DATA_BLOCK "IMAC_VALVE_I/O"
TITLE =
AUTHOR : Hottendo
FAMILY : IMAC
VERSION : 0.2


  STRUCT
   VALVE_001_ACOM : WORD ;	//VALVE - Instance 001 : 'AUTO' Mode  Command Interface
   VALVE_001_STAT : WORD ;	//                       'AUTO' Mode  Status Interface
   VALVE_00l_OSSTAT : WORD ;	//                       OS Status Word
   VALVE_00l_OSALARM : WORD ;	//                       OS Alarm Word
   VALVE_001_OSCOM : WORD ;	//                       OS Command Interface
   VALVE_002_ACOM : WORD ;	//VALVE - Instance 002 : 'AUTO' Mode  Command Interface
   VALVE_002_STAT : WORD ;	//                       'AUTO' Mode  Status Interface
   VALVE_002_OSSTAT : WORD ;	//                       OS Status Word
   VALVE_002_OSALARM : WORD ;	//                       OS Alarm Word
   VALVE_002_OSCOM : WORD ;	//                       OS Command Interface
   VALVE_003_ACOM : WORD ;	//VALVE - Instance 003 : 'AUTO' Mode  Command Interface
   VALVE_003_STAT : WORD ;	//                       'AUTO' Mode  Status Interface
   VALVE_003_OSSTAT : WORD ;	//                       OS Status Word
   VALVE_003_OSALARM : WORD ;	//                       OS Alarm Word
   VALVE_003_OSCOM : WORD ;	//                       OS Command Interface
   VALVE_004_ACOM : WORD ;	//VALVE - Instance 004 : 'AUTO' Mode  Command Interface
   VALVE_004_STAT : WORD ;	//                       'AUTO' Mode  Status Interface
   VALVE_004_OSSTAT : WORD ;	//                       OS Status Word
   VALVE_004_OSALARM : WORD ;	//                       OS Alarm Word
   VALVE_004_OSCOM : WORD ;	//                       OS Command Interface
   VALVE_005_ACOM : WORD ;	//VALVE - Instance 005 : 'AUTO' Mode  Command Interface
   VALVE_005_STAT : WORD ;	//                       'AUTO' Mode  Status Interface
   VALVE_005_OSSTAT : WORD ;	//                       OS Status Word
   VALVE_005_OSALARM : WORD ;	//                       OS Alarm Word
   VALVE_005_OSCOM : WORD ;	//                       OS Command Interface
   VALVE_006_ACOM : WORD ;	//VALVE - Instance 006 : 'AUTO' Mode  Command Interface
   VALVE_006_STAT : WORD ;	//                       'AUTO' Mode  Status Interface
   VALVE_006_OSSTAT : WORD ;	//                       OS Status Word
   VALVE_006_OSALARM : WORD ;	//                       OS Alarm Word
   VALVE_006_OSCOM : WORD ;	//                       OS Command Interface
   VALVE_007_ACOM : WORD ;	//VALVE - Instance 007 : 'AUTO' Mode  Command Interface
   VALVE_007_STAT : WORD ;	//                       'AUTO' Mode  Status Interface
   VALVE_007_OSSTAT : WORD ;	//                       OS Status Word
   VALVE_007_OSALARM : WORD ;	//                       OS Alarm Word
   VALVE_007_OSCOM : WORD ;	//                       OS Command Interface
   VALVE_008_ACOM : WORD ;	//VALVE - Instance 008 : 'AUTO' Mode  Command Interface
   VALVE_008_STAT : WORD ;	//                       'AUTO' Mode  Status Interface
   VALVE_008_OSSTAT : WORD ;	//                       OS Status Word
   VALVE_008_OSALARM : WORD ;	//                       OS Alarm Word
   VALVE_008_OSCOM : WORD ;	//                       OS Command Interface
   VALVE_009_ACOM : WORD ;	//VALVE - Instance 009 : 'AUTO' Mode  Command Interface
   VALVE_009_STAT : WORD ;	//                       'AUTO' Mode  Status Interface
   VALVE_009_OSSTAT : WORD ;	//                       OS Status Word
   VALVE_009_OSALARM : WORD ;	//                       OS Alarm Word
   VALVE_009_OSCOM : WORD ;	//                       OS Command Interface
   VALVE_010_ACOM : WORD ;	//VALVE - Instance 010 : 'AUTO' Mode  Command Interface
   VALVE_010_STAT : WORD ;	//                       'AUTO' Mode  Status Interface
   VALVE_010_OSSTAT : WORD ;	//                       OS Status Word
   VALVE_010_OSALARM : WORD ;	//                       OS Alarm Word
   VALVE_010_OSCOM : WORD ;	//                       OS Command Interface
   VALVE_011_ACOM : WORD ;	//VALVE - Instance 011 : 'AUTO' Mode  Command Interface
   VALVE_011_STAT : WORD ;	//                       'AUTO' Mode  Status Interface
   VALVE_01l_OSSTAT : WORD ;	//                       OS Status Word
   VALVE_01l_OSALARM : WORD ;	//                       OS Alarm Word
   VALVE_011_OSCOM : WORD ;	//                       OS Command Interface
   VALVE_012_ACOM : WORD ;	//VALVE - Instance 012 : 'AUTO' Mode  Command Interface
   VALVE_012_STAT : WORD ;	//                       'AUTO' Mode  Status Interface
   VALVE_012_OSSTAT : WORD ;	//                       OS Status Word
   VALVE_012_OSALARM : WORD ;	//                       OS Alarm Word
   VALVE_012_OSCOM : WORD ;	//                       OS Command Interface
   VALVE_013_ACOM : WORD ;	//VALVE - Instance 013 : 'AUTO' Mode  Command Interface
   VALVE_013_STAT : WORD ;	//                       'AUTO' Mode  Status Interface
   VALVE_013_OSSTAT : WORD ;	//                       OS Status Word
   VALVE_013_OSALARM : WORD ;	//                       OS Alarm Word
   VALVE_013_OSCOM : WORD ;	//                       OS Command Interface
   VALVE_014_ACOM : WORD ;	//VALVE - Instance 014 : 'AUTO' Mode  Command Interface
   VALVE_014_STAT : WORD ;	//                       'AUTO' Mode  Status Interface
   VALVE_014_OSSTAT : WORD ;	//                       OS Status Word
   VALVE_014_OSALARM : WORD ;	//                       OS Alarm Word
   VALVE_014_OSCOM : WORD ;	//                       OS Command Interface
   VALVE_015_ACOM : WORD ;	//VALVE - Instance 015 : 'AUTO' Mode  Command Interface
   VALVE_015_STAT : WORD ;	//                       'AUTO' Mode  Status Interface
   VALVE_015_OSSTAT : WORD ;	//                       OS Status Word
   VALVE_015_OSALARM : WORD ;	//                       OS Alarm Word
   VALVE_015_OSCOM : WORD ;	//                       OS Command Interface
   VALVE_016_ACOM : WORD ;	//VALVE - Instance 016 : 'AUTO' Mode  Command Interface
   VALVE_016_STAT : WORD ;	//                       'AUTO' Mode  Status Interface
   VALVE_016_OSSTAT : WORD ;	//                       OS Status Word
   VALVE_016_OSALARM : WORD ;	//                       OS Alarm Word
   VALVE_016_OSCOM : WORD ;	//                       OS Command Interface
   VALVE_017_ACOM : WORD ;	//VALVE - Instance 017 : 'AUTO' Mode  Command Interface
   VALVE_017_STAT : WORD ;	//                       'AUTO' Mode  Status Interface
   VALVE_017_OSSTAT : WORD ;	//                       OS Status Word
   VALVE_017_OSALARM : WORD ;	//                       OS Alarm Word
   VALVE_017_OSCOM : WORD ;	//                       OS Command Interface
   VALVE_018_ACOM : WORD ;	//VALVE - Instance 018 : 'AUTO' Mode  Command Interface
   VALVE_018_STAT : WORD ;	//                       'AUTO' Mode  Status Interface
   VALVE_018_OSSTAT : WORD ;	//                       OS Status Word
   VALVE_018_OSALARM : WORD ;	//                       OS Alarm Word
   VALVE_018_OSCOM : WORD ;	//                       OS Command Interface
   VALVE_019_ACOM : WORD ;	//VALVE - Instance 019 : 'AUTO' Mode  Command Interface
   VALVE_019_STAT : WORD ;	//                       'AUTO' Mode  Status Interface
   VALVE_019_OSSTAT : WORD ;	//                       OS Status Word
   VALVE_019_OSALARM : WORD ;	//                       OS Alarm Word
   VALVE_019_OSCOM : WORD ;	//                       OS Command Interface
   VALVE_020_ACOM : WORD ;	//VALVE - Instance 020 : 'AUTO' Mode  Command Interface
   VALVE_020_STAT : WORD ;	//                       'AUTO' Mode  Status Interface
   VALVE_020_OSSTAT : WORD ;	//                       OS Status Word
   VALVE_020_OSALARM : WORD ;	//                       OS Alarm Word
   VALVE_020_OSCOM : WORD ;	//                       OS Command Interface
   VALVE_021_ACOM : WORD ;	//VALVE - Instance 021 : 'AUTO' Mode  Command Interface
   VALVE_021_STAT : WORD ;	//                       'AUTO' Mode  Status Interface
   VALVE_02l_OSSTAT : WORD ;	//                       OS Status Word
   VALVE_02l_OSALARM : WORD ;	//                       OS Alarm Word
   VALVE_021_OSCOM : WORD ;	//                       OS Command Interface
   VALVE_022_ACOM : WORD ;	//VALVE - Instance 022 : 'AUTO' Mode  Command Interface
   VALVE_022_STAT : WORD ;	//                       'AUTO' Mode  Status Interface
   VALVE_022_OSSTAT : WORD ;	//                       OS Status Word
   VALVE_022_OSALARM : WORD ;	//                       OS Alarm Word
   VALVE_022_OSCOM : WORD ;	//                       OS Command Interface
   VALVE_023_ACOM : WORD ;	//VALVE - Instance 023 : 'AUTO' Mode  Command Interface
   VALVE_023_STAT : WORD ;	//                       'AUTO' Mode  Status Interface
   VALVE_023_OSSTAT : WORD ;	//                       OS Status Word
   VALVE_023_OSALARM : WORD ;	//                       OS Alarm Word
   VALVE_023_OSCOM : WORD ;	//                       OS Command Interface
   VALVE_024_ACOM : WORD ;	//VALVE - Instance 024 : 'AUTO' Mode  Command Interface
   VALVE_024_STAT : WORD ;	//                       'AUTO' Mode  Status Interface
   VALVE_024_OSSTAT : WORD ;	//                       OS Status Word
   VALVE_024_OSALARM : WORD ;	//                       OS Alarm Word
   VALVE_024_OSCOM : WORD ;	//                       OS Command Interface
   VALVE_025_ACOM : WORD ;	//VALVE - Instance 025 : 'AUTO' Mode  Command Interface
   VALVE_025_STAT : WORD ;	//                       'AUTO' Mode  Status Interface
   VALVE_025_OSSTAT : WORD ;	//                       OS Status Word
   VALVE_025_OSALARM : WORD ;	//                       OS Alarm Word
   VALVE_025_OSCOM : WORD ;	//                       OS Command Interface
   VALVE_026_ACOM : WORD ;	//VALVE - Instance 026 : 'AUTO' Mode  Command Interface
   VALVE_026_STAT : WORD ;	//                       'AUTO' Mode  Status Interface
   VALVE_026_OSSTAT : WORD ;	//                       OS Status Word
   VALVE_026_OSALARM : WORD ;	//                       OS Alarm Word
   VALVE_026_OSCOM : WORD ;	//                       OS Command Interface
   VALVE_027_ACOM : WORD ;	//VALVE - Instance 027 : 'AUTO' Mode  Command Interface
   VALVE_027_STAT : WORD ;	//                       'AUTO' Mode  Status Interface
   VALVE_027_OSSTAT : WORD ;	//                       OS Status Word
   VALVE_027_OSALARM : WORD ;	//                       OS Alarm Word
   VALVE_027_OSCOM : WORD ;	//                       OS Command Interface
   VALVE_028_ACOM : WORD ;	//VALVE - Instance 028 : 'AUTO' Mode  Command Interface
   VALVE_028_STAT : WORD ;	//                       'AUTO' Mode  Status Interface
   VALVE_028_OSSTAT : WORD ;	//                       OS Status Word
   VALVE_028_OSALARM : WORD ;	//                       OS Alarm Word
   VALVE_028_OSCOM : WORD ;	//                       OS Command Interface
   VALVE_029_ACOM : WORD ;	//VALVE - Instance 029 : 'AUTO' Mode  Command Interface
   VALVE_029_STAT : WORD ;	//                       'AUTO' Mode  Status Interface
   VALVE_029_OSSTAT : WORD ;	//                       OS Status Word
   VALVE_029_OSALARM : WORD ;	//                       OS Alarm Word
   VALVE_029_OSCOM : WORD ;	//                       OS Command Interface
   VALVE_030_ACOM : WORD ;	//VALVE - Instance 030 : 'AUTO' Mode  Command Interface
   VALVE_030_STAT : WORD ;	//                       'AUTO' Mode  Status Interface
   VALVE_030_OSSTAT : WORD ;	//                       OS Status Word
   VALVE_030_OSALARM : WORD ;	//                       OS Alarm Word
   VALVE_030_OSCOM : WORD ;	//                       OS Command Interface
   VALVE_031_ACOM : WORD ;	//VALVE - Instance 031 : 'AUTO' Mode  Command Interface
   VALVE_031_STAT : WORD ;	//                       'AUTO' Mode  Status Interface
   VALVE_03l_OSSTAT : WORD ;	//                       OS Status Word
   VALVE_03l_OSALARM : WORD ;	//                       OS Alarm Word
   VALVE_031_OSCOM : WORD ;	//                       OS Command Interface
   VALVE_032_ACOM : WORD ;	//VALVE - Instance 032 : 'AUTO' Mode  Command Interface
   VALVE_032_STAT : WORD ;	//                       'AUTO' Mode  Status Interface
   VALVE_032_OSSTAT : WORD ;	//                       OS Status Word
   VALVE_032_OSALARM : WORD ;	//                       OS Alarm Word
   VALVE_032_OSCOM : WORD ;	//                       OS Command Interface
   VALVE_033_ACOM : WORD ;	//VALVE - Instance 033 : 'AUTO' Mode  Command Interface
   VALVE_033_STAT : WORD ;	//                       'AUTO' Mode  Status Interface
   VALVE_033_OSSTAT : WORD ;	//                       OS Status Word
   VALVE_033_OSALARM : WORD ;	//                       OS Alarm Word
   VALVE_033_OSCOM : WORD ;	//                       OS Command Interface
   VALVE_034_ACOM : WORD ;	//VALVE - Instance 034 : 'AUTO' Mode  Command Interface
   VALVE_034_STAT : WORD ;	//                       'AUTO' Mode  Status Interface
   VALVE_034_OSSTAT : WORD ;	//                       OS Status Word
   VALVE_034_OSALARM : WORD ;	//                       OS Alarm Word
   VALVE_034_OSCOM : WORD ;	//                       OS Command Interface
   VALVE_035_ACOM : WORD ;	//VALVE - Instance 035 : 'AUTO' Mode  Command Interface
   VALVE_035_STAT : WORD ;	//                       'AUTO' Mode  Status Interface
   VALVE_035_OSSTAT : WORD ;	//                       OS Status Word
   VALVE_035_OSALARM : WORD ;	//                       OS Alarm Word
   VALVE_035_OSCOM : WORD ;	//                       OS Command Interface
   VALVE_036_ACOM : WORD ;	//VALVE - Instance 036 : 'AUTO' Mode  Command Interface
   VALVE_036_STAT : WORD ;	//                       'AUTO' Mode  Status Interface
   VALVE_036_OSSTAT : WORD ;	//                       OS Status Word
   VALVE_036_OSALARM : WORD ;	//                       OS Alarm Word
   VALVE_036_OSCOM : WORD ;	//                       OS Command Interface
   VALVE_037_ACOM : WORD ;	//VALVE - Instance 037 : 'AUTO' Mode  Command Interface
   VALVE_037_STAT : WORD ;	//                       'AUTO' Mode  Status Interface
   VALVE_037_OSSTAT : WORD ;	//                       OS Status Word
   VALVE_037_OSALARM : WORD ;	//                       OS Alarm Word
   VALVE_037_OSCOM : WORD ;	//                       OS Command Interface
   VALVE_038_ACOM : WORD ;	//VALVE - Instance 038 : 'AUTO' Mode  Command Interface
   VALVE_038_STAT : WORD ;	//                       'AUTO' Mode  Status Interface
   VALVE_038_OSSTAT : WORD ;	//                       OS Status Word
   VALVE_038_OSALARM : WORD ;	//                       OS Alarm Word
   VALVE_038_OSCOM : WORD ;	//                       OS Command Interface
   VALVE_039_ACOM : WORD ;	//VALVE - Instance 039 : 'AUTO' Mode  Command Interface
   VALVE_039_STAT : WORD ;	//                       'AUTO' Mode  Status Interface
   VALVE_039_OSSTAT : WORD ;	//                       OS Status Word
   VALVE_039_OSALARM : WORD ;	//                       OS Alarm Word
   VALVE_039_OSCOM : WORD ;	//                       OS Command Interface
   VALVE_040_ACOM : WORD ;	//VALVE - Instance 040 : 'AUTO' Mode  Command Interface
   VALVE_040_STAT : WORD ;	//                       'AUTO' Mode  Status Interface
   VALVE_040_OSSTAT : WORD ;	//                       OS Status Word
   VALVE_040_OSALARM : WORD ;	//                       OS Alarm Word
   VALVE_040_OSCOM : WORD ;	//                       OS Command Interface
   VALVE_041_ACOM : WORD ;	//VALVE - Instance 041 : 'AUTO' Mode  Command Interface
   VALVE_041_STAT : WORD ;	//                       'AUTO' Mode  Status Interface
   VALVE_04l_OSSTAT : WORD ;	//                       OS Status Word
   VALVE_04l_OSALARM : WORD ;	//                       OS Alarm Word
   VALVE_041_OSCOM : WORD ;	//                       OS Command Interface
   VALVE_042_ACOM : WORD ;	//VALVE - Instance 042 : 'AUTO' Mode  Command Interface
   VALVE_042_STAT : WORD ;	//                       'AUTO' Mode  Status Interface
   VALVE_042_OSSTAT : WORD ;	//                       OS Status Word
   VALVE_042_OSALARM : WORD ;	//                       OS Alarm Word
   VALVE_042_OSCOM : WORD ;	//                       OS Command Interface
   VALVE_043_ACOM : WORD ;	//VALVE - Instance 043 : 'AUTO' Mode  Command Interface
   VALVE_043_STAT : WORD ;	//                       'AUTO' Mode  Status Interface
   VALVE_043_OSSTAT : WORD ;	//                       OS Status Word
   VALVE_043_OSALARM : WORD ;	//                       OS Alarm Word
   VALVE_043_OSCOM : WORD ;	//                       OS Command Interface
   VALVE_044_ACOM : WORD ;	//VALVE - Instance 044 : 'AUTO' Mode  Command Interface
   VALVE_044_STAT : WORD ;	//                       'AUTO' Mode  Status Interface
   VALVE_044_OSSTAT : WORD ;	//                       OS Status Word
   VALVE_044_OSALARM : WORD ;	//                       OS Alarm Word
   VALVE_044_OSCOM : WORD ;	//                       OS Command Interface
   VALVE_045_ACOM : WORD ;	//VALVE - Instance 045 : 'AUTO' Mode  Command Interface
   VALVE_045_STAT : WORD ;	//                       'AUTO' Mode  Status Interface
   VALVE_045_OSSTAT : WORD ;	//                       OS Status Word
   VALVE_045_OSALARM : WORD ;	//                       OS Alarm Word
   VALVE_045_OSCOM : WORD ;	//                       OS Command Interface
   VALVE_046_ACOM : WORD ;	//VALVE - Instance 046 : 'AUTO' Mode  Command Interface
   VALVE_046_STAT : WORD ;	//                       'AUTO' Mode  Status Interface
   VALVE_046_OSSTAT : WORD ;	//                       OS Status Word
   VALVE_046_OSALARM : WORD ;	//                       OS Alarm Word
   VALVE_046_OSCOM : WORD ;	//                       OS Command Interface
   VALVE_047_ACOM : WORD ;	//VALVE - Instance 047 : 'AUTO' Mode  Command Interface
   VALVE_047_STAT : WORD ;	//                       'AUTO' Mode  Status Interface
   VALVE_047_OSSTAT : WORD ;	//                       OS Status Word
   VALVE_047_OSALARM : WORD ;	//                       OS Alarm Word
   VALVE_047_OSCOM : WORD ;	//                       OS Command Interface
   VALVE_048_ACOM : WORD ;	//VALVE - Instance 048 : 'AUTO' Mode  Command Interface
   VALVE_048_STAT : WORD ;	//                       'AUTO' Mode  Status Interface
   VALVE_048_OSSTAT : WORD ;	//                       OS Status Word
   VALVE_048_OSALARM : WORD ;	//                       OS Alarm Word
   VALVE_048_OSCOM : WORD ;	//                       OS Command Interface
   VALVE_049_ACOM : WORD ;	//VALVE - Instance 049 : 'AUTO' Mode  Command Interface
   VALVE_049_STAT : WORD ;	//                       'AUTO' Mode  Status Interface
   VALVE_049_OSSTAT : WORD ;	//                       OS Status Word
   VALVE_049_OSALARM : WORD ;	//                       OS Alarm Word
   VALVE_049_OSCOM : WORD ;	//                       OS Command Interface
   VALVE_050_ACOM : WORD ;	//VALVE - Instance 050 : 'AUTO' Mode  Command Interface
   VALVE_050_STAT : WORD ;	//                       'AUTO' Mode  Status Interface
   VALVE_050_OSSTAT : WORD ;	//                       OS Status Word
   VALVE_050_OSALARM : WORD ;	//                       OS Alarm Word
   VALVE_050_OSCOM : WORD ;	//                       OS Command Interface
   VALVE_051_ACOM : WORD ;	//VALVE - Instance 051 : 'AUTO' Mode  Command Interface
   VALVE_051_STAT : WORD ;	//                       'AUTO' Mode  Status Interface
   VALVE_05l_OSSTAT : WORD ;	//                       OS Status Word
   VALVE_05l_OSALARM : WORD ;	//                       OS Alarm Word
   VALVE_051_OSCOM : WORD ;	//                       OS Command Interface
   VALVE_052_ACOM : WORD ;	//VALVE - Instance 052 : 'AUTO' Mode  Command Interface
   VALVE_052_STAT : WORD ;	//                       'AUTO' Mode  Status Interface
   VALVE_052_OSSTAT : WORD ;	//                       OS Status Word
   VALVE_052_OSALARM : WORD ;	//                       OS Alarm Word
   VALVE_052_OSCOM : WORD ;	//                       OS Command Interface
   VALVE_053_ACOM : WORD ;	//VALVE - Instance 053 : 'AUTO' Mode  Command Interface
   VALVE_053_STAT : WORD ;	//                       'AUTO' Mode  Status Interface
   VALVE_053_OSSTAT : WORD ;	//                       OS Status Word
   VALVE_053_OSALARM : WORD ;	//                       OS Alarm Word
   VALVE_053_OSCOM : WORD ;	//                       OS Command Interface
   VALVE_054_ACOM : WORD ;	//VALVE - Instance 054 : 'AUTO' Mode  Command Interface
   VALVE_054_STAT : WORD ;	//                       'AUTO' Mode  Status Interface
   VALVE_054_OSSTAT : WORD ;	//                       OS Status Word
   VALVE_054_OSALARM : WORD ;	//                       OS Alarm Word
   VALVE_054_OSCOM : WORD ;	//                       OS Command Interface
   VALVE_055_ACOM : WORD ;	//VALVE - Instance 055 : 'AUTO' Mode  Command Interface
   VALVE_055_STAT : WORD ;	//                       'AUTO' Mode  Status Interface
   VALVE_055_OSSTAT : WORD ;	//                       OS Status Word
   VALVE_055_OSALARM : WORD ;	//                       OS Alarm Word
   VALVE_055_OSCOM : WORD ;	//                       OS Command Interface
   VALVE_056_ACOM : WORD ;	//VALVE - Instance 056 : 'AUTO' Mode  Command Interface
   VALVE_056_STAT : WORD ;	//                       'AUTO' Mode  Status Interface
   VALVE_056_OSSTAT : WORD ;	//                       OS Status Word
   VALVE_056_OSALARM : WORD ;	//                       OS Alarm Word
   VALVE_056_OSCOM : WORD ;	//                       OS Command Interface
   VALVE_057_ACOM : WORD ;	//VALVE - Instance 057 : 'AUTO' Mode  Command Interface
   VALVE_057_STAT : WORD ;	//                       'AUTO' Mode  Status Interface
   VALVE_057_OSSTAT : WORD ;	//                       OS Status Word
   VALVE_057_OSALARM : WORD ;	//                       OS Alarm Word
   VALVE_057_OSCOM : WORD ;	//                       OS Command Interface
   VALVE_058_ACOM : WORD ;	//VALVE - Instance 058 : 'AUTO' Mode  Command Interface
   VALVE_058_STAT : WORD ;	//                       'AUTO' Mode  Status Interface
   VALVE_058_OSSTAT : WORD ;	//                       OS Status Word
   VALVE_058_OSALARM : WORD ;	//                       OS Alarm Word
   VALVE_058_OSCOM : WORD ;	//                       OS Command Interface
   VALVE_059_ACOM : WORD ;	//VALVE - Instance 059 : 'AUTO' Mode  Command Interface
   VALVE_059_STAT : WORD ;	//                       'AUTO' Mode  Status Interface
   VALVE_059_OSSTAT : WORD ;	//                       OS Status Word
   VALVE_059_OSALARM : WORD ;	//                       OS Alarm Word
   VALVE_059_OSCOM : WORD ;	//                       OS Command Interface
   VALVE_060_ACOM : WORD ;	//VALVE - Instance 060 : 'AUTO' Mode  Command Interface
   VALVE_060_STAT : WORD ;	//                       'AUTO' Mode  Status Interface
   VALVE_060_OSSTAT : WORD ;	//                       OS Status Word
   VALVE_060_OSALARM : WORD ;	//                       OS Alarm Word
   VALVE_060_OSCOM : WORD ;	//                       OS Command Interface
   VALVE_061_ACOM : WORD ;	//VALVE - Instance 061 : 'AUTO' Mode  Command Interface
   VALVE_061_STAT : WORD ;	//                       'AUTO' Mode  Status Interface
   VALVE_06l_OSSTAT : WORD ;	//                       OS Status Word
   VALVE_06l_OSALARM : WORD ;	//                       OS Alarm Word
   VALVE_061_OSCOM : WORD ;	//                       OS Command Interface
   VALVE_062_ACOM : WORD ;	//VALVE - Instance 062 : 'AUTO' Mode  Command Interface
   VALVE_062_STAT : WORD ;	//                       'AUTO' Mode  Status Interface
   VALVE_062_OSSTAT : WORD ;	//                       OS Status Word
   VALVE_062_OSALARM : WORD ;	//                       OS Alarm Word
   VALVE_062_OSCOM : WORD ;	//                       OS Command Interface
   VALVE_063_ACOM : WORD ;	//VALVE - Instance 063 : 'AUTO' Mode  Command Interface
   VALVE_063_STAT : WORD ;	//                       'AUTO' Mode  Status Interface
   VALVE_063_OSSTAT : WORD ;	//                       OS Status Word
   VALVE_063_OSALARM : WORD ;	//                       OS Alarm Word
   VALVE_063_OSCOM : WORD ;	//                       OS Command Interface
   VALVE_064_ACOM : WORD ;	//VALVE - Instance 064 : 'AUTO' Mode  Command Interface
   VALVE_064_STAT : WORD ;	//                       'AUTO' Mode  Status Interface
   VALVE_064_OSSTAT : WORD ;	//                       OS Status Word
   VALVE_064_OSALARM : WORD ;	//                       OS Alarm Word
   VALVE_064_OSCOM : WORD ;	//                       OS Command Interface
   VALVE_065_ACOM : WORD ;	//VALVE - Instance 065 : 'AUTO' Mode  Command Interface
   VALVE_065_STAT : WORD ;	//                       'AUTO' Mode  Status Interface
   VALVE_065_OSSTAT : WORD ;	//                       OS Status Word
   VALVE_065_OSALARM : WORD ;	//                       OS Alarm Word
   VALVE_065_OSCOM : WORD ;	//                       OS Command Interface
   VALVE_066_ACOM : WORD ;	//VALVE - Instance 066 : 'AUTO' Mode  Command Interface
   VALVE_066_STAT : WORD ;	//                       'AUTO' Mode  Status Interface
   VALVE_066_OSSTAT : WORD ;	//                       OS Status Word
   VALVE_066_OSALARM : WORD ;	//                       OS Alarm Word
   VALVE_066_OSCOM : WORD ;	//                       OS Command Interface
   VALVE_067_ACOM : WORD ;	//VALVE - Instance 067 : 'AUTO' Mode  Command Interface
   VALVE_067_STAT : WORD ;	//                       'AUTO' Mode  Status Interface
   VALVE_067_OSSTAT : WORD ;	//                       OS Status Word
   VALVE_067_OSALARM : WORD ;	//                       OS Alarm Word
   VALVE_067_OSCOM : WORD ;	//                       OS Command Interface
   VALVE_068_ACOM : WORD ;	//VALVE - Instance 068 : 'AUTO' Mode  Command Interface
   VALVE_068_STAT : WORD ;	//                       'AUTO' Mode  Status Interface
   VALVE_068_OSSTAT : WORD ;	//                       OS Status Word
   VALVE_068_OSALARM : WORD ;	//                       OS Alarm Word
   VALVE_068_OSCOM : WORD ;	//                       OS Command Interface
   VALVE_069_ACOM : WORD ;	//VALVE - Instance 069 : 'AUTO' Mode  Command Interface
   VALVE_069_STAT : WORD ;	//                       'AUTO' Mode  Status Interface
   VALVE_069_OSSTAT : WORD ;	//                       OS Status Word
   VALVE_069_OSALARM : WORD ;	//                       OS Alarm Word
   VALVE_069_OSCOM : WORD ;	//                       OS Command Interface
   VALVE_070_ACOM : WORD ;	//VALVE - Instance 070 : 'AUTO' Mode  Command Interface
   VALVE_070_STAT : WORD ;	//                       'AUTO' Mode  Status Interface
   VALVE_070_OSSTAT : WORD ;	//                       OS Status Word
   VALVE_070_OSALARM : WORD ;	//                       OS Alarm Word
   VALVE_070_OSCOM : WORD ;	//                       OS Command Interface
   VALVE_071_ACOM : WORD ;	//VALVE - Instance 071 : 'AUTO' Mode  Command Interface
   VALVE_071_STAT : WORD ;	//                       'AUTO' Mode  Status Interface
   VALVE_07l_OSSTAT : WORD ;	//                       OS Status Word
   VALVE_07l_OSALARM : WORD ;	//                       OS Alarm Word
   VALVE_071_OSCOM : WORD ;	//                       OS Command Interface
   VALVE_072_ACOM : WORD ;	//VALVE - Instance 072 : 'AUTO' Mode  Command Interface
   VALVE_072_STAT : WORD ;	//                       'AUTO' Mode  Status Interface
   VALVE_072_OSSTAT : WORD ;	//                       OS Status Word
   VALVE_072_OSALARM : WORD ;	//                       OS Alarm Word
   VALVE_072_OSCOM : WORD ;	//                       OS Command Interface
   VALVE_073_ACOM : WORD ;	//VALVE - Instance 073 : 'AUTO' Mode  Command Interface
   VALVE_073_STAT : WORD ;	//                       'AUTO' Mode  Status Interface
   VALVE_073_OSSTAT : WORD ;	//                       OS Status Word
   VALVE_073_OSALARM : WORD ;	//                       OS Alarm Word
   VALVE_073_OSCOM : WORD ;	//                       OS Command Interface
   VALVE_074_ACOM : WORD ;	//VALVE - Instance 074 : 'AUTO' Mode  Command Interface
   VALVE_074_STAT : WORD ;	//                       'AUTO' Mode  Status Interface
   VALVE_074_OSSTAT : WORD ;	//                       OS Status Word
   VALVE_074_OSALARM : WORD ;	//                       OS Alarm Word
   VALVE_074_OSCOM : WORD ;	//                       OS Command Interface
   VALVE_075_ACOM : WORD ;	//VALVE - Instance 075 : 'AUTO' Mode  Command Interface
   VALVE_075_STAT : WORD ;	//                       'AUTO' Mode  Status Interface
   VALVE_075_OSSTAT : WORD ;	//                       OS Status Word
   VALVE_075_OSALARM : WORD ;	//                       OS Alarm Word
   VALVE_075_OSCOM : WORD ;	//                       OS Command Interface
   VALVE_076_ACOM : WORD ;	//VALVE - Instance 076 : 'AUTO' Mode  Command Interface
   VALVE_076_STAT : WORD ;	//                       'AUTO' Mode  Status Interface
   VALVE_076_OSSTAT : WORD ;	//                       OS Status Word
   VALVE_076_OSALARM : WORD ;	//                       OS Alarm Word
   VALVE_076_OSCOM : WORD ;	//                       OS Command Interface
   VALVE_077_ACOM : WORD ;	//VALVE - Instance 077 : 'AUTO' Mode  Command Interface
   VALVE_077_STAT : WORD ;	//                       'AUTO' Mode  Status Interface
   VALVE_077_OSSTAT : WORD ;	//                       OS Status Word
   VALVE_077_OSALARM : WORD ;	//                       OS Alarm Word
   VALVE_077_OSCOM : WORD ;	//                       OS Command Interface
   VALVE_078_ACOM : WORD ;	//VALVE - Instance 078 : 'AUTO' Mode  Command Interface
   VALVE_078_STAT : WORD ;	//                       'AUTO' Mode  Status Interface
   VALVE_078_OSSTAT : WORD ;	//                       OS Status Word
   VALVE_078_OSALARM : WORD ;	//                       OS Alarm Word
   VALVE_078_OSCOM : WORD ;	//                       OS Command Interface
   VALVE_079_ACOM : WORD ;	//VALVE - Instance 079 : 'AUTO' Mode  Command Interface
   VALVE_079_STAT : WORD ;	//                       'AUTO' Mode  Status Interface
   VALVE_079_OSSTAT : WORD ;	//                       OS Status Word
   VALVE_079_OSALARM : WORD ;	//                       OS Alarm Word
   VALVE_079_OSCOM : WORD ;	//                       OS Command Interface
   VALVE_080_ACOM : WORD ;	//VALVE - Instance 080 : 'AUTO' Mode  Command Interface
   VALVE_080_STAT : WORD ;	//                       'AUTO' Mode  Status Interface
   VALVE_080_OSSTAT : WORD ;	//                       OS Status Word
   VALVE_080_OSALARM : WORD ;	//                       OS Alarm Word
   VALVE_080_OSCOM : WORD ;	//                       OS Command Interface
   VALVE_081_ACOM : WORD ;	//VALVE - Instance 081 : 'AUTO' Mode  Command Interface
   VALVE_081_STAT : WORD ;	//                       'AUTO' Mode  Status Interface
   VALVE_08l_OSSTAT : WORD ;	//                       OS Status Word
   VALVE_08l_OSALARM : WORD ;	//                       OS Alarm Word
   VALVE_081_OSCOM : WORD ;	//                       OS Command Interface
   VALVE_082_ACOM : WORD ;	//VALVE - Instance 082 : 'AUTO' Mode  Command Interface
   VALVE_082_STAT : WORD ;	//                       'AUTO' Mode  Status Interface
   VALVE_082_OSSTAT : WORD ;	//                       OS Status Word
   VALVE_082_OSALARM : WORD ;	//                       OS Alarm Word
   VALVE_082_OSCOM : WORD ;	//                       OS Command Interface
   VALVE_083_ACOM : WORD ;	//VALVE - Instance 083 : 'AUTO' Mode  Command Interface
   VALVE_083_STAT : WORD ;	//                       'AUTO' Mode  Status Interface
   VALVE_083_OSSTAT : WORD ;	//                       OS Status Word
   VALVE_083_OSALARM : WORD ;	//                       OS Alarm Word
   VALVE_083_OSCOM : WORD ;	//                       OS Command Interface
   VALVE_084_ACOM : WORD ;	//VALVE - Instance 084 : 'AUTO' Mode  Command Interface
   VALVE_084_STAT : WORD ;	//                       'AUTO' Mode  Status Interface
   VALVE_084_OSSTAT : WORD ;	//                       OS Status Word
   VALVE_084_OSALARM : WORD ;	//                       OS Alarm Word
   VALVE_084_OSCOM : WORD ;	//                       OS Command Interface
   VALVE_085_ACOM : WORD ;	//VALVE - Instance 085 : 'AUTO' Mode  Command Interface
   VALVE_085_STAT : WORD ;	//                       'AUTO' Mode  Status Interface
   VALVE_085_OSSTAT : WORD ;	//                       OS Status Word
   VALVE_085_OSALARM : WORD ;	//                       OS Alarm Word
   VALVE_085_OSCOM : WORD ;	//                       OS Command Interface
   VALVE_086_ACOM : WORD ;	//VALVE - Instance 086 : 'AUTO' Mode  Command Interface
   VALVE_086_STAT : WORD ;	//                       'AUTO' Mode  Status Interface
   VALVE_086_OSSTAT : WORD ;	//                       OS Status Word
   VALVE_086_OSALARM : WORD ;	//                       OS Alarm Word
   VALVE_086_OSCOM : WORD ;	//                       OS Command Interface
   VALVE_087_ACOM : WORD ;	//VALVE - Instance 087 : 'AUTO' Mode  Command Interface
   VALVE_087_STAT : WORD ;	//                       'AUTO' Mode  Status Interface
   VALVE_087_OSSTAT : WORD ;	//                       OS Status Word
   VALVE_087_OSALARM : WORD ;	//                       OS Alarm Word
   VALVE_087_OSCOM : WORD ;	//                       OS Command Interface
   VALVE_088_ACOM : WORD ;	//VALVE - Instance 088 : 'AUTO' Mode  Command Interface
   VALVE_088_STAT : WORD ;	//                       'AUTO' Mode  Status Interface
   VALVE_088_OSSTAT : WORD ;	//                       OS Status Word
   VALVE_088_OSALARM : WORD ;	//                       OS Alarm Word
   VALVE_088_OSCOM : WORD ;	//                       OS Command Interface
   VALVE_089_ACOM : WORD ;	//VALVE - Instance 089 : 'AUTO' Mode  Command Interface
   VALVE_089_STAT : WORD ;	//                       'AUTO' Mode  Status Interface
   VALVE_089_OSSTAT : WORD ;	//                       OS Status Word
   VALVE_089_OSALARM : WORD ;	//                       OS Alarm Word
   VALVE_089_OSCOM : WORD ;	//                       OS Command Interface
   VALVE_090_ACOM : WORD ;	//VALVE - Instance 090 : 'AUTO' Mode  Command Interface
   VALVE_090_STAT : WORD ;	//                       'AUTO' Mode  Status Interface
   VALVE_090_OSSTAT : WORD ;	//                       OS Status Word
   VALVE_090_OSALARM : WORD ;	//                       OS Alarm Word
   VALVE_090_OSCOM : WORD ;	//                       OS Command Interface
   VALVE_091_ACOM : WORD ;	//VALVE - Instance 091 : 'AUTO' Mode  Command Interface
   VALVE_091_STAT : WORD ;	//                       'AUTO' Mode  Status Interface
   VALVE_09l_OSSTAT : WORD ;	//                       OS Status Word
   VALVE_09l_OSALARM : WORD ;	//                       OS Alarm Word
   VALVE_091_OSCOM : WORD ;	//                       OS Command Interface
   VALVE_092_ACOM : WORD ;	//VALVE - Instance 092 : 'AUTO' Mode  Command Interface
   VALVE_092_STAT : WORD ;	//                       'AUTO' Mode  Status Interface
   VALVE_092_OSSTAT : WORD ;	//                       OS Status Word
   VALVE_092_OSALARM : WORD ;	//                       OS Alarm Word
   VALVE_092_OSCOM : WORD ;	//                       OS Command Interface
   VALVE_093_ACOM : WORD ;	//VALVE - Instance 093 : 'AUTO' Mode  Command Interface
   VALVE_093_STAT : WORD ;	//                       'AUTO' Mode  Status Interface
   VALVE_093_OSSTAT : WORD ;	//                       OS Status Word
   VALVE_093_OSALARM : WORD ;	//                       OS Alarm Word
   VALVE_093_OSCOM : WORD ;	//                       OS Command Interface
   VALVE_094_ACOM : WORD ;	//VALVE - Instance 094 : 'AUTO' Mode  Command Interface
   VALVE_094_STAT : WORD ;	//                       'AUTO' Mode  Status Interface
   VALVE_094_OSSTAT : WORD ;	//                       OS Status Word
   VALVE_094_OSALARM : WORD ;	//                       OS Alarm Word
   VALVE_094_OSCOM : WORD ;	//                       OS Command Interface
   VALVE_095_ACOM : WORD ;	//VALVE - Instance 095 : 'AUTO' Mode  Command Interface
   VALVE_095_STAT : WORD ;	//                       'AUTO' Mode  Status Interface
   VALVE_095_OSSTAT : WORD ;	//                       OS Status Word
   VALVE_095_OSALARM : WORD ;	//                       OS Alarm Word
   VALVE_095_OSCOM : WORD ;	//                       OS Command Interface
   VALVE_096_ACOM : WORD ;	//VALVE - Instance 096 : 'AUTO' Mode  Command Interface
   VALVE_096_STAT : WORD ;	//                       'AUTO' Mode  Status Interface
   VALVE_096_OSSTAT : WORD ;	//                       OS Status Word
   VALVE_096_OSALARM : WORD ;	//                       OS Alarm Word
   VALVE_096_OSCOM : WORD ;	//                       OS Command Interface
   VALVE_097_ACOM : WORD ;	//VALVE - Instance 097 : 'AUTO' Mode  Command Interface
   VALVE_097_STAT : WORD ;	//                       'AUTO' Mode  Status Interface
   VALVE_097_OSSTAT : WORD ;	//                       OS Status Word
   VALVE_097_OSALARM : WORD ;	//                       OS Alarm Word
   VALVE_097_OSCOM : WORD ;	//                       OS Command Interface
   VALVE_098_ACOM : WORD ;	//VALVE - Instance 098 : 'AUTO' Mode  Command Interface
   VALVE_098_STAT : WORD ;	//                       'AUTO' Mode  Status Interface
   VALVE_098_OSSTAT : WORD ;	//                       OS Status Word
   VALVE_098_OSALARM : WORD ;	//                       OS Alarm Word
   VALVE_098_OSCOM : WORD ;	//                       OS Command Interface
   VALVE_099_ACOM : WORD ;	//VALVE - Instance 099 : 'AUTO' Mode  Command Interface
   VALVE_099_STAT : WORD ;	//                       'AUTO' Mode  Status Interface
   VALVE_099_OSSTAT : WORD ;	//                       OS Status Word
   VALVE_099_OSALARM : WORD ;	//                       OS Alarm Word
   VALVE_099_OSCOM : WORD ;	//                       OS Command Interface
   VALVE_100_ACOM : WORD ;	//VALVE - Instance 100 : 'AUTO' Mode  Command Interface
   VALVE_100_STAT : WORD ;	//                       'AUTO' Mode  Status Interface
   VALVE_100_OSSTAT : WORD ;	//                       OS Status Word
   VALVE_100_OSALARM : WORD ;	//                       OS Alarm Word
   VALVE_100_OSCOM : WORD ;	//                       OS Command Interface
   VALVE_100_ACOM1 : WORD ;	//VALVE - Instance 100 : 'AUTO' Mode  Command Interface
   VALVE_100_STAT1 : WORD ;	//                       'AUTO' Mode  Status Interface
   VALVE_100_OSSTAT1 : WORD ;	//                       OS Status Word
   VALVE_100_OSALARM1 : WORD ;	//                       OS Alarm Word
   VALVE_100_OSCOM1 : WORD ;	//                       OS Command Interface
  END_STRUCT ;
BEGIN
   VALVE_001_ACOM := W#16#0;
   VALVE_001_STAT := W#16#0;
   VALVE_00l_OSSTAT := W#16#0;
   VALVE_00l_OSALARM := W#16#0;
   VALVE_001_OSCOM := W#16#0;
   VALVE_002_ACOM := W#16#0;
   VALVE_002_STAT := W#16#0;
   VALVE_002_OSSTAT := W#16#0;
   VALVE_002_OSALARM := W#16#0;
   VALVE_002_OSCOM := W#16#0;
   VALVE_003_ACOM := W#16#0;
   VALVE_003_STAT := W#16#0;
   VALVE_003_OSSTAT := W#16#0;
   VALVE_003_OSALARM := W#16#0;
   VALVE_003_OSCOM := W#16#0;
   VALVE_004_ACOM := W#16#0;
   VALVE_004_STAT := W#16#0;
   VALVE_004_OSSTAT := W#16#0;
   VALVE_004_OSALARM := W#16#0;
   VALVE_004_OSCOM := W#16#0;
   VALVE_005_ACOM := W#16#0;
   VALVE_005_STAT := W#16#0;
   VALVE_005_OSSTAT := W#16#0;
   VALVE_005_OSALARM := W#16#0;
   VALVE_005_OSCOM := W#16#0;
   VALVE_006_ACOM := W#16#0;
   VALVE_006_STAT := W#16#0;
   VALVE_006_OSSTAT := W#16#0;
   VALVE_006_OSALARM := W#16#0;
   VALVE_006_OSCOM := W#16#0;
   VALVE_007_ACOM := W#16#0;
   VALVE_007_STAT := W#16#0;
   VALVE_007_OSSTAT := W#16#0;
   VALVE_007_OSALARM := W#16#0;
   VALVE_007_OSCOM := W#16#0;
   VALVE_008_ACOM := W#16#0;
   VALVE_008_STAT := W#16#0;
   VALVE_008_OSSTAT := W#16#0;
   VALVE_008_OSALARM := W#16#0;
   VALVE_008_OSCOM := W#16#0;
   VALVE_009_ACOM := W#16#0;
   VALVE_009_STAT := W#16#0;
   VALVE_009_OSSTAT := W#16#0;
   VALVE_009_OSALARM := W#16#0;
   VALVE_009_OSCOM := W#16#0;
   VALVE_010_ACOM := W#16#0;
   VALVE_010_STAT := W#16#0;
   VALVE_010_OSSTAT := W#16#0;
   VALVE_010_OSALARM := W#16#0;
   VALVE_010_OSCOM := W#16#0;
   VALVE_011_ACOM := W#16#0;
   VALVE_011_STAT := W#16#0;
   VALVE_01l_OSSTAT := W#16#0;
   VALVE_01l_OSALARM := W#16#0;
   VALVE_011_OSCOM := W#16#0;
   VALVE_012_ACOM := W#16#0;
   VALVE_012_STAT := W#16#0;
   VALVE_012_OSSTAT := W#16#0;
   VALVE_012_OSALARM := W#16#0;
   VALVE_012_OSCOM := W#16#0;
   VALVE_013_ACOM := W#16#0;
   VALVE_013_STAT := W#16#0;
   VALVE_013_OSSTAT := W#16#0;
   VALVE_013_OSALARM := W#16#0;
   VALVE_013_OSCOM := W#16#0;
   VALVE_014_ACOM := W#16#0;
   VALVE_014_STAT := W#16#0;
   VALVE_014_OSSTAT := W#16#0;
   VALVE_014_OSALARM := W#16#0;
   VALVE_014_OSCOM := W#16#0;
   VALVE_015_ACOM := W#16#0;
   VALVE_015_STAT := W#16#0;
   VALVE_015_OSSTAT := W#16#0;
   VALVE_015_OSALARM := W#16#0;
   VALVE_015_OSCOM := W#16#0;
   VALVE_016_ACOM := W#16#0;
   VALVE_016_STAT := W#16#0;
   VALVE_016_OSSTAT := W#16#0;
   VALVE_016_OSALARM := W#16#0;
   VALVE_016_OSCOM := W#16#0;
   VALVE_017_ACOM := W#16#0;
   VALVE_017_STAT := W#16#0;
   VALVE_017_OSSTAT := W#16#0;
   VALVE_017_OSALARM := W#16#0;
   VALVE_017_OSCOM := W#16#0;
   VALVE_018_ACOM := W#16#0;
   VALVE_018_STAT := W#16#0;
   VALVE_018_OSSTAT := W#16#0;
   VALVE_018_OSALARM := W#16#0;
   VALVE_018_OSCOM := W#16#0;
   VALVE_019_ACOM := W#16#0;
   VALVE_019_STAT := W#16#0;
   VALVE_019_OSSTAT := W#16#0;
   VALVE_019_OSALARM := W#16#0;
   VALVE_019_OSCOM := W#16#0;
   VALVE_020_ACOM := W#16#0;
   VALVE_020_STAT := W#16#0;
   VALVE_020_OSSTAT := W#16#0;
   VALVE_020_OSALARM := W#16#0;
   VALVE_020_OSCOM := W#16#0;
   VALVE_021_ACOM := W#16#0;
   VALVE_021_STAT := W#16#0;
   VALVE_02l_OSSTAT := W#16#0;
   VALVE_02l_OSALARM := W#16#0;
   VALVE_021_OSCOM := W#16#0;
   VALVE_022_ACOM := W#16#0;
   VALVE_022_STAT := W#16#0;
   VALVE_022_OSSTAT := W#16#0;
   VALVE_022_OSALARM := W#16#0;
   VALVE_022_OSCOM := W#16#0;
   VALVE_023_ACOM := W#16#0;
   VALVE_023_STAT := W#16#0;
   VALVE_023_OSSTAT := W#16#0;
   VALVE_023_OSALARM := W#16#0;
   VALVE_023_OSCOM := W#16#0;
   VALVE_024_ACOM := W#16#0;
   VALVE_024_STAT := W#16#0;
   VALVE_024_OSSTAT := W#16#0;
   VALVE_024_OSALARM := W#16#0;
   VALVE_024_OSCOM := W#16#0;
   VALVE_025_ACOM := W#16#0;
   VALVE_025_STAT := W#16#0;
   VALVE_025_OSSTAT := W#16#0;
   VALVE_025_OSALARM := W#16#0;
   VALVE_025_OSCOM := W#16#0;
   VALVE_026_ACOM := W#16#0;
   VALVE_026_STAT := W#16#0;
   VALVE_026_OSSTAT := W#16#0;
   VALVE_026_OSALARM := W#16#0;
   VALVE_026_OSCOM := W#16#0;
   VALVE_027_ACOM := W#16#0;
   VALVE_027_STAT := W#16#0;
   VALVE_027_OSSTAT := W#16#0;
   VALVE_027_OSALARM := W#16#0;
   VALVE_027_OSCOM := W#16#0;
   VALVE_028_ACOM := W#16#0;
   VALVE_028_STAT := W#16#0;
   VALVE_028_OSSTAT := W#16#0;
   VALVE_028_OSALARM := W#16#0;
   VALVE_028_OSCOM := W#16#0;
   VALVE_029_ACOM := W#16#0;
   VALVE_029_STAT := W#16#0;
   VALVE_029_OSSTAT := W#16#0;
   VALVE_029_OSALARM := W#16#0;
   VALVE_029_OSCOM := W#16#0;
   VALVE_030_ACOM := W#16#0;
   VALVE_030_STAT := W#16#0;
   VALVE_030_OSSTAT := W#16#0;
   VALVE_030_OSALARM := W#16#0;
   VALVE_030_OSCOM := W#16#0;
   VALVE_031_ACOM := W#16#0;
   VALVE_031_STAT := W#16#0;
   VALVE_03l_OSSTAT := W#16#0;
   VALVE_03l_OSALARM := W#16#0;
   VALVE_031_OSCOM := W#16#0;
   VALVE_032_ACOM := W#16#0;
   VALVE_032_STAT := W#16#0;
   VALVE_032_OSSTAT := W#16#0;
   VALVE_032_OSALARM := W#16#0;
   VALVE_032_OSCOM := W#16#0;
   VALVE_033_ACOM := W#16#0;
   VALVE_033_STAT := W#16#0;
   VALVE_033_OSSTAT := W#16#0;
   VALVE_033_OSALARM := W#16#0;
   VALVE_033_OSCOM := W#16#0;
   VALVE_034_ACOM := W#16#0;
   VALVE_034_STAT := W#16#0;
   VALVE_034_OSSTAT := W#16#0;
   VALVE_034_OSALARM := W#16#0;
   VALVE_034_OSCOM := W#16#0;
   VALVE_035_ACOM := W#16#0;
   VALVE_035_STAT := W#16#0;
   VALVE_035_OSSTAT := W#16#0;
   VALVE_035_OSALARM := W#16#0;
   VALVE_035_OSCOM := W#16#0;
   VALVE_036_ACOM := W#16#0;
   VALVE_036_STAT := W#16#0;
   VALVE_036_OSSTAT := W#16#0;
   VALVE_036_OSALARM := W#16#0;
   VALVE_036_OSCOM := W#16#0;
   VALVE_037_ACOM := W#16#0;
   VALVE_037_STAT := W#16#0;
   VALVE_037_OSSTAT := W#16#0;
   VALVE_037_OSALARM := W#16#0;
   VALVE_037_OSCOM := W#16#0;
   VALVE_038_ACOM := W#16#0;
   VALVE_038_STAT := W#16#0;
   VALVE_038_OSSTAT := W#16#0;
   VALVE_038_OSALARM := W#16#0;
   VALVE_038_OSCOM := W#16#0;
   VALVE_039_ACOM := W#16#0;
   VALVE_039_STAT := W#16#0;
   VALVE_039_OSSTAT := W#16#0;
   VALVE_039_OSALARM := W#16#0;
   VALVE_039_OSCOM := W#16#0;
   VALVE_040_ACOM := W#16#0;
   VALVE_040_STAT := W#16#0;
   VALVE_040_OSSTAT := W#16#0;
   VALVE_040_OSALARM := W#16#0;
   VALVE_040_OSCOM := W#16#0;
   VALVE_041_ACOM := W#16#0;
   VALVE_041_STAT := W#16#0;
   VALVE_04l_OSSTAT := W#16#0;
   VALVE_04l_OSALARM := W#16#0;
   VALVE_041_OSCOM := W#16#0;
   VALVE_042_ACOM := W#16#0;
   VALVE_042_STAT := W#16#0;
   VALVE_042_OSSTAT := W#16#0;
   VALVE_042_OSALARM := W#16#0;
   VALVE_042_OSCOM := W#16#0;
   VALVE_043_ACOM := W#16#0;
   VALVE_043_STAT := W#16#0;
   VALVE_043_OSSTAT := W#16#0;
   VALVE_043_OSALARM := W#16#0;
   VALVE_043_OSCOM := W#16#0;
   VALVE_044_ACOM := W#16#0;
   VALVE_044_STAT := W#16#0;
   VALVE_044_OSSTAT := W#16#0;
   VALVE_044_OSALARM := W#16#0;
   VALVE_044_OSCOM := W#16#0;
   VALVE_045_ACOM := W#16#0;
   VALVE_045_STAT := W#16#0;
   VALVE_045_OSSTAT := W#16#0;
   VALVE_045_OSALARM := W#16#0;
   VALVE_045_OSCOM := W#16#0;
   VALVE_046_ACOM := W#16#0;
   VALVE_046_STAT := W#16#0;
   VALVE_046_OSSTAT := W#16#0;
   VALVE_046_OSALARM := W#16#0;
   VALVE_046_OSCOM := W#16#0;
   VALVE_047_ACOM := W#16#0;
   VALVE_047_STAT := W#16#0;
   VALVE_047_OSSTAT := W#16#0;
   VALVE_047_OSALARM := W#16#0;
   VALVE_047_OSCOM := W#16#0;
   VALVE_048_ACOM := W#16#0;
   VALVE_048_STAT := W#16#0;
   VALVE_048_OSSTAT := W#16#0;
   VALVE_048_OSALARM := W#16#0;
   VALVE_048_OSCOM := W#16#0;
   VALVE_049_ACOM := W#16#0;
   VALVE_049_STAT := W#16#0;
   VALVE_049_OSSTAT := W#16#0;
   VALVE_049_OSALARM := W#16#0;
   VALVE_049_OSCOM := W#16#0;
   VALVE_050_ACOM := W#16#0;
   VALVE_050_STAT := W#16#0;
   VALVE_050_OSSTAT := W#16#0;
   VALVE_050_OSALARM := W#16#0;
   VALVE_050_OSCOM := W#16#0;
   VALVE_051_ACOM := W#16#0;
   VALVE_051_STAT := W#16#0;
   VALVE_05l_OSSTAT := W#16#0;
   VALVE_05l_OSALARM := W#16#0;
   VALVE_051_OSCOM := W#16#0;
   VALVE_052_ACOM := W#16#0;
   VALVE_052_STAT := W#16#0;
   VALVE_052_OSSTAT := W#16#0;
   VALVE_052_OSALARM := W#16#0;
   VALVE_052_OSCOM := W#16#0;
   VALVE_053_ACOM := W#16#0;
   VALVE_053_STAT := W#16#0;
   VALVE_053_OSSTAT := W#16#0;
   VALVE_053_OSALARM := W#16#0;
   VALVE_053_OSCOM := W#16#0;
   VALVE_054_ACOM := W#16#0;
   VALVE_054_STAT := W#16#0;
   VALVE_054_OSSTAT := W#16#0;
   VALVE_054_OSALARM := W#16#0;
   VALVE_054_OSCOM := W#16#0;
   VALVE_055_ACOM := W#16#0;
   VALVE_055_STAT := W#16#0;
   VALVE_055_OSSTAT := W#16#0;
   VALVE_055_OSALARM := W#16#0;
   VALVE_055_OSCOM := W#16#0;
   VALVE_056_ACOM := W#16#0;
   VALVE_056_STAT := W#16#0;
   VALVE_056_OSSTAT := W#16#0;
   VALVE_056_OSALARM := W#16#0;
   VALVE_056_OSCOM := W#16#0;
   VALVE_057_ACOM := W#16#0;
   VALVE_057_STAT := W#16#0;
   VALVE_057_OSSTAT := W#16#0;
   VALVE_057_OSALARM := W#16#0;
   VALVE_057_OSCOM := W#16#0;
   VALVE_058_ACOM := W#16#0;
   VALVE_058_STAT := W#16#0;
   VALVE_058_OSSTAT := W#16#0;
   VALVE_058_OSALARM := W#16#0;
   VALVE_058_OSCOM := W#16#0;
   VALVE_059_ACOM := W#16#0;
   VALVE_059_STAT := W#16#0;
   VALVE_059_OSSTAT := W#16#0;
   VALVE_059_OSALARM := W#16#0;
   VALVE_059_OSCOM := W#16#0;
   VALVE_060_ACOM := W#16#0;
   VALVE_060_STAT := W#16#0;
   VALVE_060_OSSTAT := W#16#0;
   VALVE_060_OSALARM := W#16#0;
   VALVE_060_OSCOM := W#16#0;
   VALVE_061_ACOM := W#16#0;
   VALVE_061_STAT := W#16#0;
   VALVE_06l_OSSTAT := W#16#0;
   VALVE_06l_OSALARM := W#16#0;
   VALVE_061_OSCOM := W#16#0;
   VALVE_062_ACOM := W#16#0;
   VALVE_062_STAT := W#16#0;
   VALVE_062_OSSTAT := W#16#0;
   VALVE_062_OSALARM := W#16#0;
   VALVE_062_OSCOM := W#16#0;
   VALVE_063_ACOM := W#16#0;
   VALVE_063_STAT := W#16#0;
   VALVE_063_OSSTAT := W#16#0;
   VALVE_063_OSALARM := W#16#0;
   VALVE_063_OSCOM := W#16#0;
   VALVE_064_ACOM := W#16#0;
   VALVE_064_STAT := W#16#0;
   VALVE_064_OSSTAT := W#16#0;
   VALVE_064_OSALARM := W#16#0;
   VALVE_064_OSCOM := W#16#0;
   VALVE_065_ACOM := W#16#0;
   VALVE_065_STAT := W#16#0;
   VALVE_065_OSSTAT := W#16#0;
   VALVE_065_OSALARM := W#16#0;
   VALVE_065_OSCOM := W#16#0;
   VALVE_066_ACOM := W#16#0;
   VALVE_066_STAT := W#16#0;
   VALVE_066_OSSTAT := W#16#0;
   VALVE_066_OSALARM := W#16#0;
   VALVE_066_OSCOM := W#16#0;
   VALVE_067_ACOM := W#16#0;
   VALVE_067_STAT := W#16#0;
   VALVE_067_OSSTAT := W#16#0;
   VALVE_067_OSALARM := W#16#0;
   VALVE_067_OSCOM := W#16#0;
   VALVE_068_ACOM := W#16#0;
   VALVE_068_STAT := W#16#0;
   VALVE_068_OSSTAT := W#16#0;
   VALVE_068_OSALARM := W#16#0;
   VALVE_068_OSCOM := W#16#0;
   VALVE_069_ACOM := W#16#0;
   VALVE_069_STAT := W#16#0;
   VALVE_069_OSSTAT := W#16#0;
   VALVE_069_OSALARM := W#16#0;
   VALVE_069_OSCOM := W#16#0;
   VALVE_070_ACOM := W#16#0;
   VALVE_070_STAT := W#16#0;
   VALVE_070_OSSTAT := W#16#0;
   VALVE_070_OSALARM := W#16#0;
   VALVE_070_OSCOM := W#16#0;
   VALVE_071_ACOM := W#16#0;
   VALVE_071_STAT := W#16#0;
   VALVE_07l_OSSTAT := W#16#0;
   VALVE_07l_OSALARM := W#16#0;
   VALVE_071_OSCOM := W#16#0;
   VALVE_072_ACOM := W#16#0;
   VALVE_072_STAT := W#16#0;
   VALVE_072_OSSTAT := W#16#0;
   VALVE_072_OSALARM := W#16#0;
   VALVE_072_OSCOM := W#16#0;
   VALVE_073_ACOM := W#16#0;
   VALVE_073_STAT := W#16#0;
   VALVE_073_OSSTAT := W#16#0;
   VALVE_073_OSALARM := W#16#0;
   VALVE_073_OSCOM := W#16#0;
   VALVE_074_ACOM := W#16#0;
   VALVE_074_STAT := W#16#0;
   VALVE_074_OSSTAT := W#16#0;
   VALVE_074_OSALARM := W#16#0;
   VALVE_074_OSCOM := W#16#0;
   VALVE_075_ACOM := W#16#0;
   VALVE_075_STAT := W#16#0;
   VALVE_075_OSSTAT := W#16#0;
   VALVE_075_OSALARM := W#16#0;
   VALVE_075_OSCOM := W#16#0;
   VALVE_076_ACOM := W#16#0;
   VALVE_076_STAT := W#16#0;
   VALVE_076_OSSTAT := W#16#0;
   VALVE_076_OSALARM := W#16#0;
   VALVE_076_OSCOM := W#16#0;
   VALVE_077_ACOM := W#16#0;
   VALVE_077_STAT := W#16#0;
   VALVE_077_OSSTAT := W#16#0;
   VALVE_077_OSALARM := W#16#0;
   VALVE_077_OSCOM := W#16#0;
   VALVE_078_ACOM := W#16#0;
   VALVE_078_STAT := W#16#0;
   VALVE_078_OSSTAT := W#16#0;
   VALVE_078_OSALARM := W#16#0;
   VALVE_078_OSCOM := W#16#0;
   VALVE_079_ACOM := W#16#0;
   VALVE_079_STAT := W#16#0;
   VALVE_079_OSSTAT := W#16#0;
   VALVE_079_OSALARM := W#16#0;
   VALVE_079_OSCOM := W#16#0;
   VALVE_080_ACOM := W#16#0;
   VALVE_080_STAT := W#16#0;
   VALVE_080_OSSTAT := W#16#0;
   VALVE_080_OSALARM := W#16#0;
   VALVE_080_OSCOM := W#16#0;
   VALVE_081_ACOM := W#16#0;
   VALVE_081_STAT := W#16#0;
   VALVE_08l_OSSTAT := W#16#0;
   VALVE_08l_OSALARM := W#16#0;
   VALVE_081_OSCOM := W#16#0;
   VALVE_082_ACOM := W#16#0;
   VALVE_082_STAT := W#16#0;
   VALVE_082_OSSTAT := W#16#0;
   VALVE_082_OSALARM := W#16#0;
   VALVE_082_OSCOM := W#16#0;
   VALVE_083_ACOM := W#16#0;
   VALVE_083_STAT := W#16#0;
   VALVE_083_OSSTAT := W#16#0;
   VALVE_083_OSALARM := W#16#0;
   VALVE_083_OSCOM := W#16#0;
   VALVE_084_ACOM := W#16#0;
   VALVE_084_STAT := W#16#0;
   VALVE_084_OSSTAT := W#16#0;
   VALVE_084_OSALARM := W#16#0;
   VALVE_084_OSCOM := W#16#0;
   VALVE_085_ACOM := W#16#0;
   VALVE_085_STAT := W#16#0;
   VALVE_085_OSSTAT := W#16#0;
   VALVE_085_OSALARM := W#16#0;
   VALVE_085_OSCOM := W#16#0;
   VALVE_086_ACOM := W#16#0;
   VALVE_086_STAT := W#16#0;
   VALVE_086_OSSTAT := W#16#0;
   VALVE_086_OSALARM := W#16#0;
   VALVE_086_OSCOM := W#16#0;
   VALVE_087_ACOM := W#16#0;
   VALVE_087_STAT := W#16#0;
   VALVE_087_OSSTAT := W#16#0;
   VALVE_087_OSALARM := W#16#0;
   VALVE_087_OSCOM := W#16#0;
   VALVE_088_ACOM := W#16#0;
   VALVE_088_STAT := W#16#0;
   VALVE_088_OSSTAT := W#16#0;
   VALVE_088_OSALARM := W#16#0;
   VALVE_088_OSCOM := W#16#0;
   VALVE_089_ACOM := W#16#0;
   VALVE_089_STAT := W#16#0;
   VALVE_089_OSSTAT := W#16#0;
   VALVE_089_OSALARM := W#16#0;
   VALVE_089_OSCOM := W#16#0;
   VALVE_090_ACOM := W#16#0;
   VALVE_090_STAT := W#16#0;
   VALVE_090_OSSTAT := W#16#0;
   VALVE_090_OSALARM := W#16#0;
   VALVE_090_OSCOM := W#16#0;
   VALVE_091_ACOM := W#16#0;
   VALVE_091_STAT := W#16#0;
   VALVE_09l_OSSTAT := W#16#0;
   VALVE_09l_OSALARM := W#16#0;
   VALVE_091_OSCOM := W#16#0;
   VALVE_092_ACOM := W#16#0;
   VALVE_092_STAT := W#16#0;
   VALVE_092_OSSTAT := W#16#0;
   VALVE_092_OSALARM := W#16#0;
   VALVE_092_OSCOM := W#16#0;
   VALVE_093_ACOM := W#16#0;
   VALVE_093_STAT := W#16#0;
   VALVE_093_OSSTAT := W#16#0;
   VALVE_093_OSALARM := W#16#0;
   VALVE_093_OSCOM := W#16#0;
   VALVE_094_ACOM := W#16#0;
   VALVE_094_STAT := W#16#0;
   VALVE_094_OSSTAT := W#16#0;
   VALVE_094_OSALARM := W#16#0;
   VALVE_094_OSCOM := W#16#0;
   VALVE_095_ACOM := W#16#0;
   VALVE_095_STAT := W#16#0;
   VALVE_095_OSSTAT := W#16#0;
   VALVE_095_OSALARM := W#16#0;
   VALVE_095_OSCOM := W#16#0;
   VALVE_096_ACOM := W#16#0;
   VALVE_096_STAT := W#16#0;
   VALVE_096_OSSTAT := W#16#0;
   VALVE_096_OSALARM := W#16#0;
   VALVE_096_OSCOM := W#16#0;
   VALVE_097_ACOM := W#16#0;
   VALVE_097_STAT := W#16#0;
   VALVE_097_OSSTAT := W#16#0;
   VALVE_097_OSALARM := W#16#0;
   VALVE_097_OSCOM := W#16#0;
   VALVE_098_ACOM := W#16#0;
   VALVE_098_STAT := W#16#0;
   VALVE_098_OSSTAT := W#16#0;
   VALVE_098_OSALARM := W#16#0;
   VALVE_098_OSCOM := W#16#0;
   VALVE_099_ACOM := W#16#0;
   VALVE_099_STAT := W#16#0;
   VALVE_099_OSSTAT := W#16#0;
   VALVE_099_OSALARM := W#16#0;
   VALVE_099_OSCOM := W#16#0;
   VALVE_100_ACOM := W#16#0;
   VALVE_100_STAT := W#16#0;
   VALVE_100_OSSTAT := W#16#0;
   VALVE_100_OSALARM := W#16#0;
   VALVE_100_OSCOM := W#16#0;
   VALVE_100_ACOM1 := W#16#0;
   VALVE_100_STAT1 := W#16#0;
   VALVE_100_OSSTAT1 := W#16#0;
   VALVE_100_OSALARM1 := W#16#0;
   VALVE_100_OSCOM1 := W#16#0;
END_DATA_BLOCK

